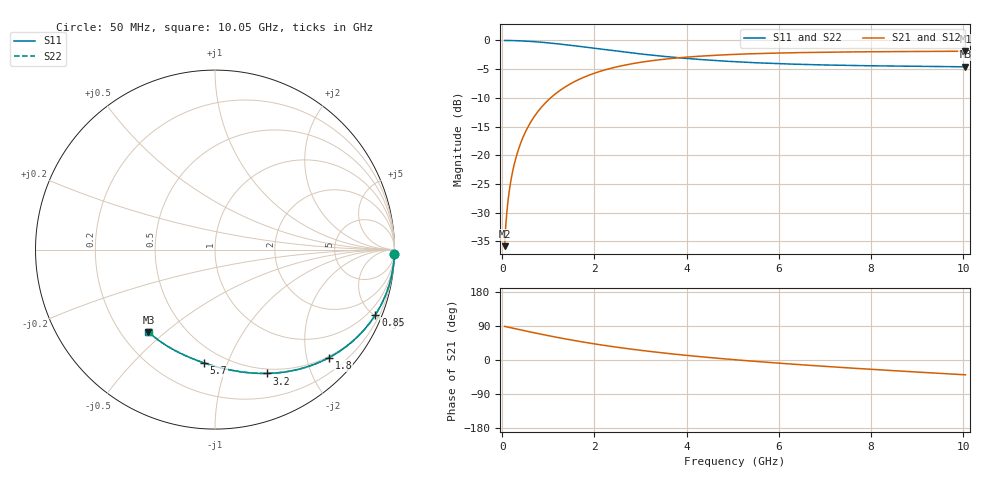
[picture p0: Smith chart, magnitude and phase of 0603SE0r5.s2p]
! AVX Thin Film Operation		Date: August 2001
! Description: Accu-P® Series, Thin Film, SMD, RF Capacitor
! Part Number: 06035J0R5ABT
! 50 MHz  -  10.05 GHz
! Serial Measurements
# mhz S db R 50
!	S11		S21		S12		S22
!	dB	Phase	dB	Phase	dB	Phase	dB	Phase
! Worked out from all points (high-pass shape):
!   401 points, 50 MHz to 10.05 GHz, reference 50 ohm
!   highest |S21| = -1.87 dB at 10.05 GHz (marker M1); lowest = -35.8 dB at 50 MHz (marker M2)
!   |S21| within 3 dB of the highest: 2.343 GHz to end of sweep
!   lowest |S11| = -4.6 dB at 10.05 GHz (marker M3), VSWR 3.87, Z = 15.6 - j22 ohm
!   |S11| at or under -10 dB: nowhere
!   |S22| runs from -4.6 to 0.0 dB; largest |S21 - S12| = 0
!   S11 on the Smith chart (normalised r, x): 50 MHz: 1, -86; 850 MHz: 0.48, -5.07; 1.8 GHz: 0.47, -2.43; 3.2 GHz: 0.45, -1.41; 5.7 GHz: 0.39, -0.83; 10.05 GHz: 0.31, -0.44
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50  -0.00 -1.3  -35.82 88.7  -35.82 88.7  -0.00 -1.3
75  -0.00 -2.0  -32.30 88.0  -32.30 88.0  -0.00 -2.0
125  -0.01 -3.3  -27.86 86.7  -27.86 86.7  -0.01 -3.3
175  -0.01 -4.7  -24.95 85.3  -24.95 85.3  -0.01 -4.7
225  -0.02 -6.0  -22.78 84.0  -22.78 84.0  -0.02 -6.0
300  -0.04 -8.0  -20.30 82.0  -20.30 82.0  -0.04 -8.0
400  -0.07 -10.6  -17.85 79.4  -17.85 79.4  -0.07 -10.6
525  -0.12 -13.9  -15.55 76.1  -15.55 76.1  -0.12 -13.9
675  -0.20 -17.7  -13.47 72.3  -13.47 72.3  -0.20 -17.7
850  -0.31 -22.1  -11.62 67.9  -11.62 67.9  -0.31 -22.1
1250  -0.63 -31.7  -8.71 58.3  -8.71 58.3  -0.63 -31.7
1725  -1.09 -42.0  -6.57 48.0  -6.57 48.0  -1.09 -42.0
1800  -1.16 -43.5  -6.31 46.5  -6.31 46.5  -1.16 -43.5
2425  -1.80 -55.1  -4.71 34.8  -4.71 34.8  -1.80 -55.1
3200  -2.52 -67.3  -3.57 22.7  -3.57 22.7  -2.52 -67.2
3400  -2.69 -70.1  -3.37 19.9  -3.37 19.9  -2.69 -70.0
4175  -3.24 -79.8  -2.80 10.1  -2.80 10.1  -3.24 -79.8
5050  -3.70 -89.3  -2.42 0.7  -2.42 0.7  -3.70 -89.2
5700  -3.95 -95.5  -2.25 -5.6  -2.25 -5.6  -3.95 -95.5
6725  -4.22 -104.5  -2.08 -14.5  -2.08 -14.5  -4.22 -104.4
8400  -4.45 -117.4  -1.95 -27.5  -1.95 -27.5  -4.45 -117.3
10050  -4.59 -128.9  -1.88 -39.1  -1.88 -39.1  -4.59 -128.9
